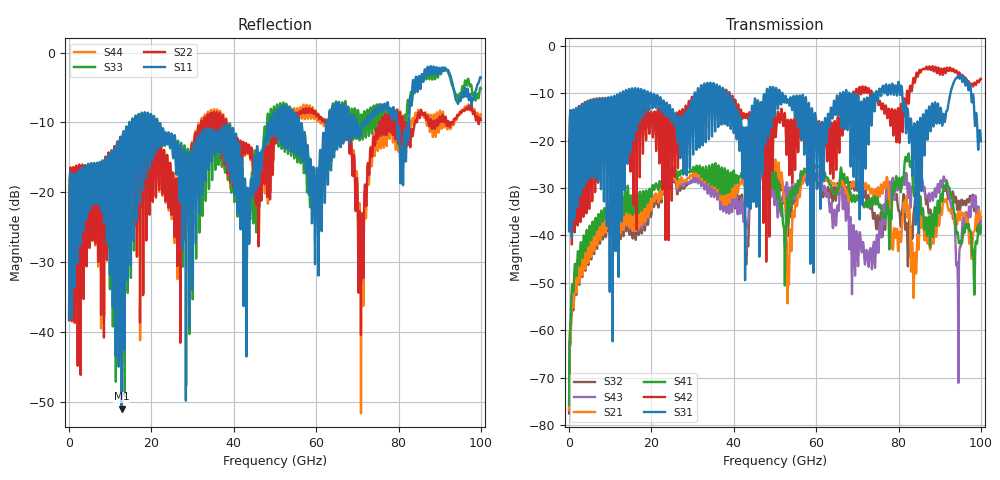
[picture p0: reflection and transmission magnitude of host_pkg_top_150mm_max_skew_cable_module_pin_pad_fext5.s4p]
# Hz S RI R 50
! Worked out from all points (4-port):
!   10000 points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, 10 MHz to 100 GHz, reference 50 ohm
!   strongest paths, dB at 10 MHz, 25.01 GHz, 50.01 GHz, 75.01 GHz, 100 GHz:
!     S31: -39.1, -14.2, -13.9, -11.7, -20.1
!     S42: -39.1, -23.6, -16.0, -11.7, -6.9
!     S41: -75.7, -25.6, -27.8, -32.7, -38.0
!     S21: -76.8, -26.9, -25.0, -29.8, -36.1
!     S43: -76.8, -27.4, -31.4, -43.3, -36.1
!     S32: -77.5, -27.9, -25.8, -35.7, -36.3
!   lowest |S11| = -51.0 dB at 12.78 GHz (marker M1), VSWR 1.01, Z = 50 + j0.281 ohm
!   |S11| at or under -10 dB: start of sweep to 14.63 GHz; 21.42 GHz to 48.86 GHz (27.44 GHz wide, 78.1 % of centre); 55.79 GHz to 62.43 GHz (6.635 GHz wide, 11.2 % of centre)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
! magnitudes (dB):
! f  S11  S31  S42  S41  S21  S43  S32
! 10 MHz  -38.3  -39.1  -39.1  -75.7  -76.8  -76.8  -77.5
! 2.49 GHz  -16.9  -13.1  -13.0  -46.4  -50.0  -48.0  -50.4
! 12.78 GHz  -51.0  -26.3  -19.2  -31.8  -33.5  -33.6  -34.5
! 64.83 GHz  -7.9  -13.4  -25.1  -31.1  -29.2  -37.8  -32.4
! 71.14 GHz  -10.0  -15.4  -8.8  -33.2  -29.4  -43.3  -30.2
! 75.67 GHz  -8.5  -10.1  -12.3  -33.9  -29.4  -37.5  -35.4
! 100 GHz  -3.5  -20.1  -6.9  -38.0  -36.1  -36.1  -36.3
